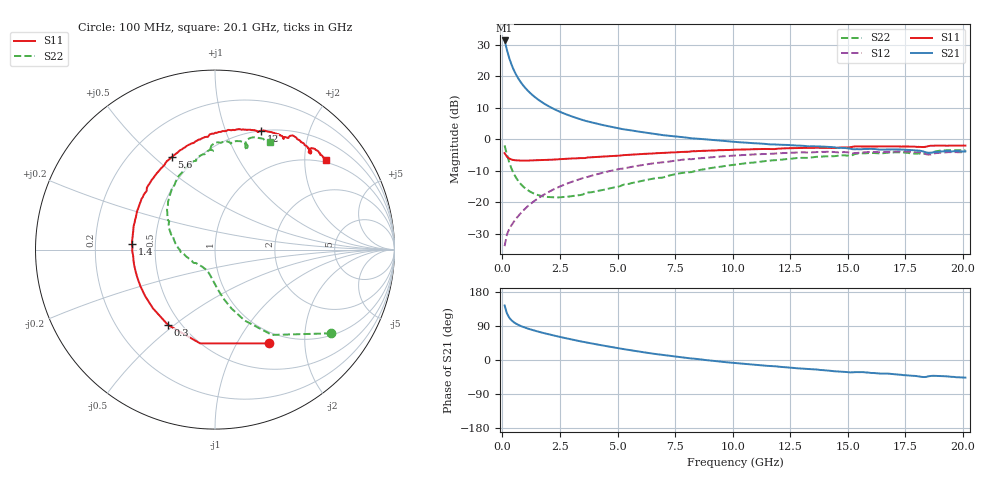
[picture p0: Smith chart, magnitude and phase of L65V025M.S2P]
!  Infineon Technologies AG
! BFR380L3 , PF131585-7, No.6, Th 09.10.01, soldered on pcb-board, measured with PP GSG850
!  Vce=5.0 V,  Ic=25.0 mA
! Common Emitter S-Parameters:  15. November 2001
#  GHz  S  MA  R  50
! f  S11  S21  S12  S22
! GHz  Mag  Ang  Mag  Ang  Mag  Ang  Mag  Ang
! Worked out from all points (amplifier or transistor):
!   201 points, 100 MHz to 20.1 GHz, reference 50 ohm
!   highest |S21| = 31.4 dB at 100 MHz (marker M1)
!   |S21| within 3 dB of that: start of sweep to 200.5 MHz
!   unconditionally stable (mu >= 1): 1.367 GHz to 4.373 GHz
!   at 3.4 GHz: K = 1.02, MAG = 8.6 dB, |S12| = -12.6 dB
!   at 10.1 GHz: K = 0.95, MSG = 2.2 dB, |S12| = -5.2 dB
!   at 20.1 GHz: K = 0.98, MSG = 0.1 dB, |S12| = -4.1 dB
!   S11 on the Smith chart (normalised r, x): 100 MHz: 0.84, -1.37; 300 MHz: 0.43, -0.47; 1.4 GHz: 0.37, +0.03; 5.6 GHz: 0.37, +0.57; 12 GHz: 0.50, +1.34; 20.1 GHz: 0.93, +2.52
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0.1  0.6023 -60.1  37.3 143.9  0.01995 64.0  0.7979 -35.8
0.2  0.5289 -99.0  26.45 123.1  0.03039 57.2  0.5718 -56.2
0.3  0.4948 -122.0  19.63 111.8  0.03748 55.0  0.4285 -67.3
0.4  0.476 -136.6  15.39 104.7  0.04296 56.1  0.3405 -74.4
0.5  0.4674 -146.5  12.59 99.6  0.04877 57.9  0.2835 -79.5
0.6  0.4627 -154.1  10.63 95.8  0.05478 59.5  0.2442 -83.4
0.7  0.4601 -160.2  9.201 92.6  0.06061 60.8  0.2155 -86.8
0.8  0.4588 -165.0  8.095 89.8  0.06673 62.0  0.1944 -89.7
1  0.4579 -172.6  6.539 85.2  0.07939 63.6  0.1655 -95.0
1.2  0.4611 -178.9  5.489 81.2  0.09215 64.3  0.1476 -99.9
1.4  0.4637 175.9  4.732 77.6  0.1053 64.6  0.1356 -104.5
1.8  0.4668 167.3  3.722 71.1  0.1316 64.3  0.1231 -113.2
2.2  0.4748 159.9  3.084 65.1  0.1578 63.0  0.1195 -122.1
2.7  0.4864 151.4  2.553 58.2  0.1901 60.8  0.1211 -132.5
3.5  0.5015 139.8  2.02 48.0  0.2417 56.3  0.1324 -145.8
5.6  0.5694 115.1  1.382 25.6  0.3634 43.0  0.2006 179.2
6.8  0.6028 103.5  1.189 14.5  0.4264 34.7  0.2437 162.9
10.1  0.6837 78.9  0.9091 -7.9  0.5512 13.2  0.3954 129.5
12  0.711 68.9  0.8207 -17.7  0.5996 1.7  0.4707 112.6
13.5  0.7283 61.3  0.7763 -24.7  0.6221 -7.7  0.5178 101.3
16.8  0.7702 48.7  0.6895 -36.1  0.6315 -23.9  0.6134 79.6
20.1  0.7951 39.1  0.6428 -46.5  0.6263 -37.8  0.6745 63.0
